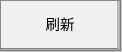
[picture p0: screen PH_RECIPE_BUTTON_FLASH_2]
VISUALIZATION PH_RECIPE_BUTTON_FLASH_2  // 122x52
VAR_IN_OUT
	RECIPE_CTRL_V2 : ST_RecipeCtrl_2;
END_VAR
    Button (0,0 120x50), "刷新", input disabled if: (RECIPE_CTRL_V2.sStatus.bBusy) <> 0, text list: 'TextList_Recipe', text index: 110
        p55702900: SEL(RECIPE_CTRL_V2.sCmd.bFlash, 16#000000, 16#00FF00)
        tap RECIPE_CTRL_V2.sCmd.bFlash
END_VISUALIZATION
